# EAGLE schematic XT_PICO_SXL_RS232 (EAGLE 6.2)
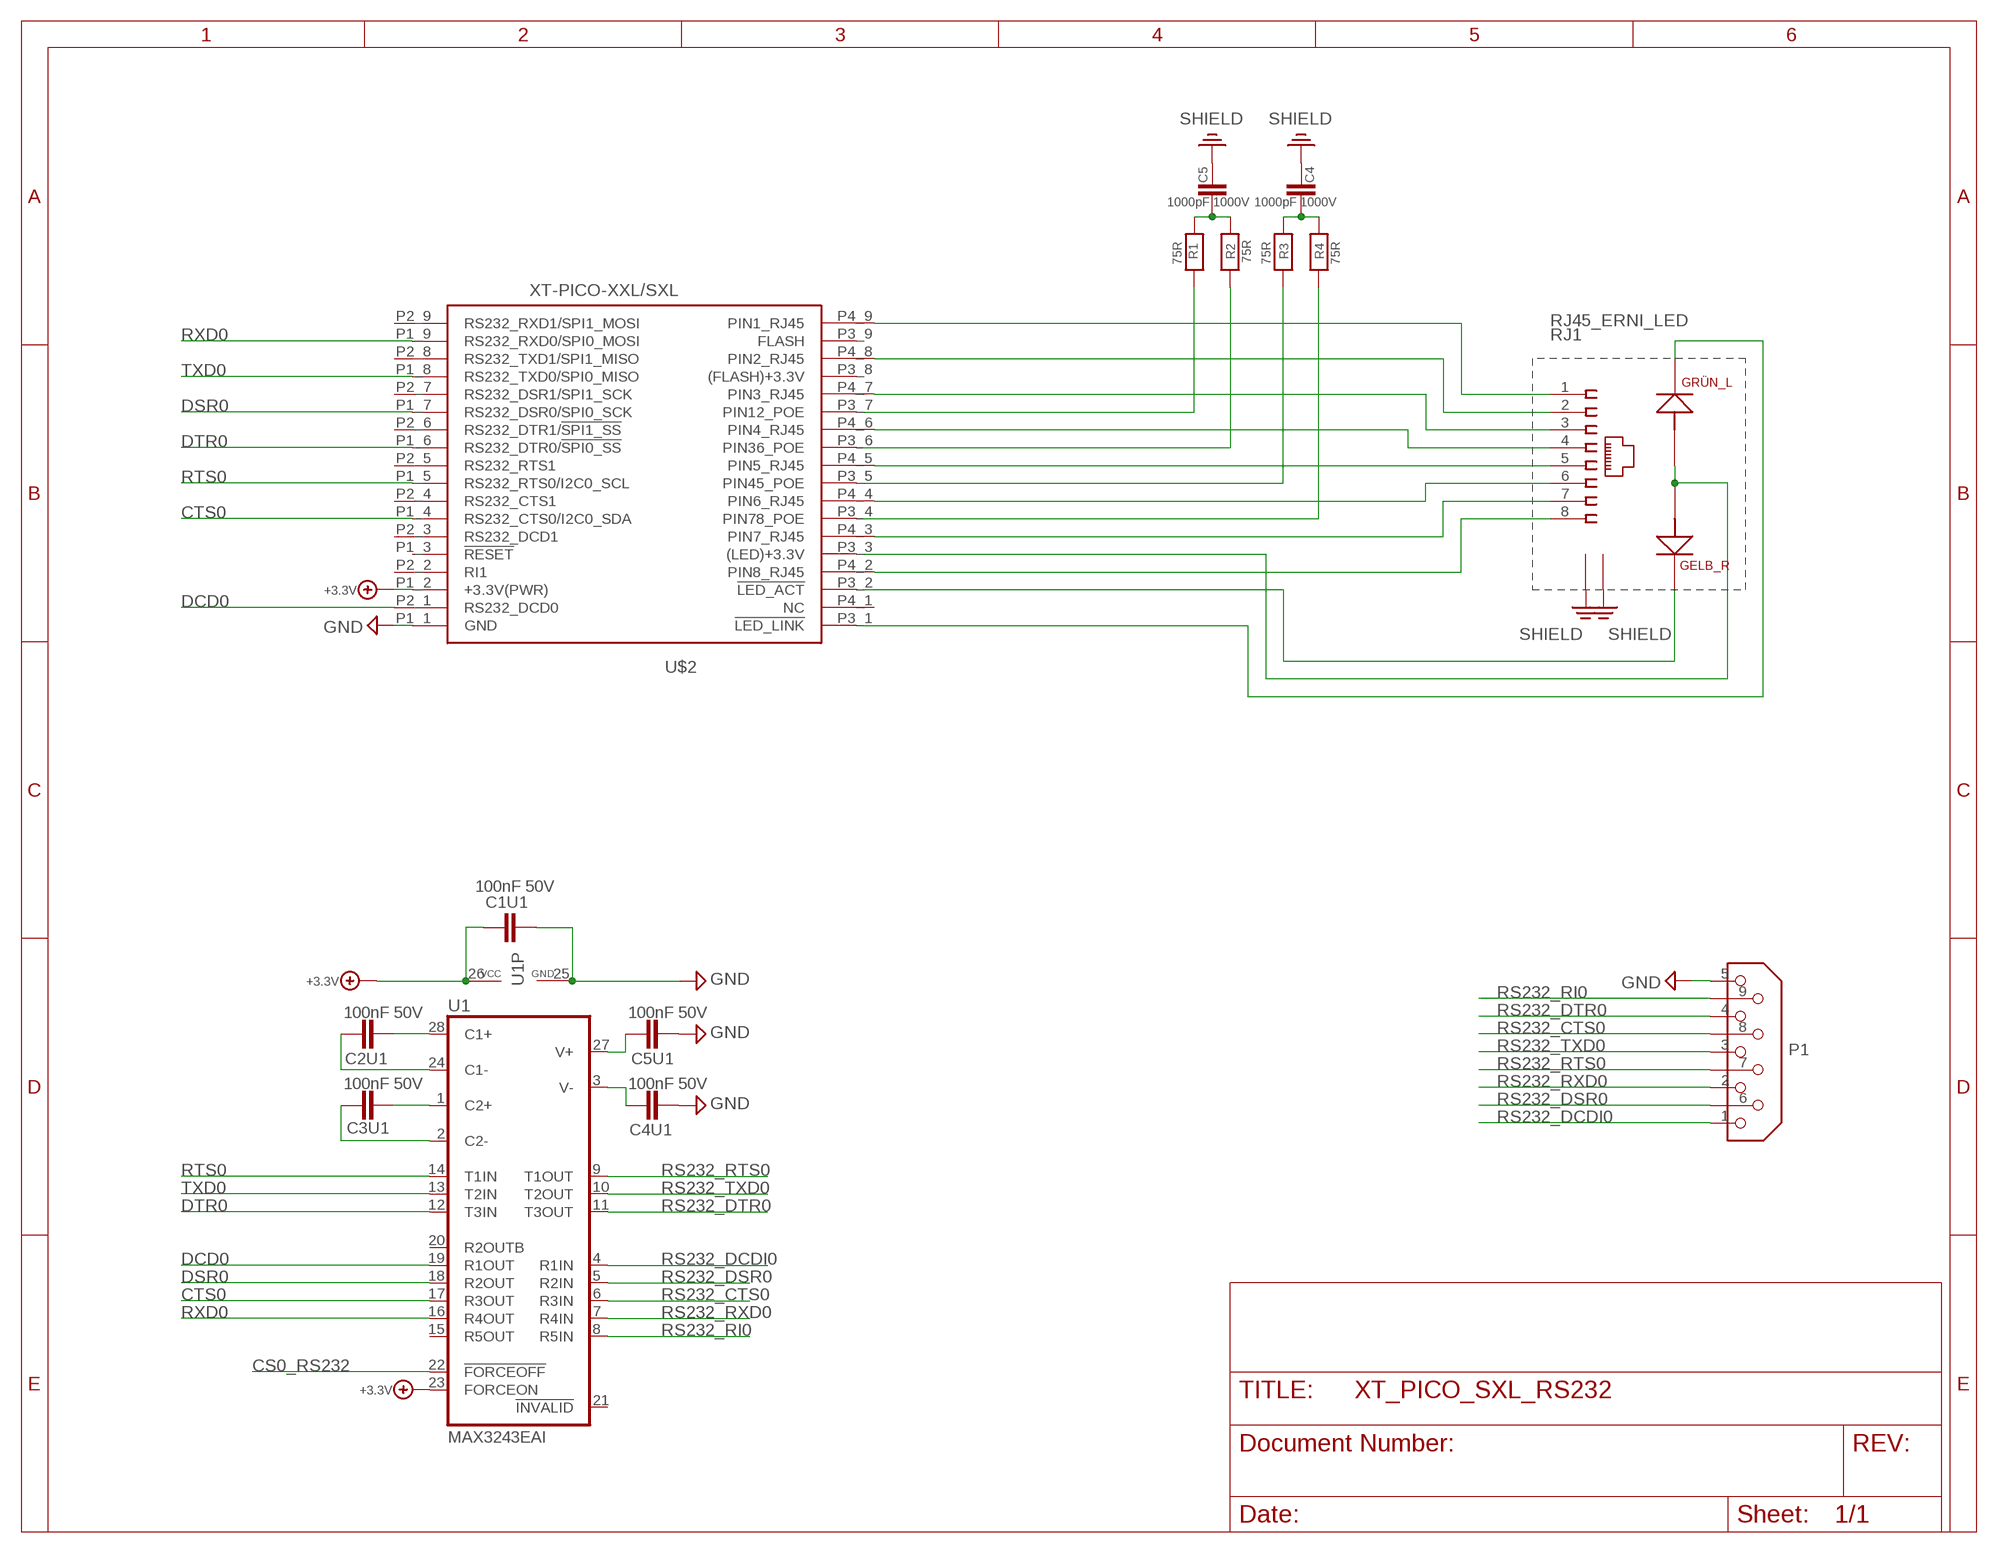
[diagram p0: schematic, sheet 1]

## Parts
C1U1  100nF 50V  CHIP-C-0603  [SMD-0603]
C2U1  100nF 50V  CHIP-C-0603  [SMD-0603]
C3U1  100nF 50V  CHIP-C-0603  [SMD-0603]
C4  1000pF 1000V  CHIP-C-1210  [SMD-1210]
C4U1  100nF 50V  CHIP-C-0603  [SMD-0603]
C5  1000pF 1000V  CHIP-C-1210  [SMD-1210]
C5U1  100nF 50V  CHIP-C-0603  [SMD-0603]
P1  DB9  [MSUB9-5]
R1  75R  CHIP-R-0603  [SMD-0603]
R2  75R  CHIP-R-0603  [SMD-0603]
R3  75R  CHIP-R-0603  [SMD-0603]
R4  75R  CHIP-R-0603  [SMD-0603]
RJ1  RJ45_ERNI_LED  [ORCAD_X_ERNI_RJ45_LED]
U1  MAX3243EAI  [SSOP28]
U$2  XT-PICO-XXL/SXL  [XT-PICO-XXL/SXL]

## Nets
+3.3V: C1U1.1 U1.23(FORCEON) U1.26(VCC) U$2.P1_2(+3.3V(PWR))
CS0_RS232: U1.22(!FORCEOFF)
CTS0: U1.17(R3OUT) U$2.P1_4(RS232_CTS0/I2C0_SDA)
DCD0: U1.19(R1OUT) U$2.P2_1(RS232_DCD0)
DSR0: U1.18(R2OUT) U$2.P1_7(RS232_DSR0/SPI0_SCK)
DTR0: U1.12(T3IN) U$2.P1_6(RS232_DTR0/!SPI0_SS!)
GND: C1U1.2 C4U1.2 C5U1.2 P1.5 U1.25(GND) U$2.P1_1(GND)
N$1: RJ1.4 U$2.P4_6(PIN4_RJ45)
N$2: RJ1.5 U$2.P4_5(PIN5_RJ45)
N$3: RJ1.7 U$2.P4_3(PIN7_RJ45)
N$4: R1.2 U$2.P3_7(PIN12_POE)
N$5: RJ1.8 U$2.P4_2(PIN8_RJ45)
N$6: R2.2 U$2.P3_6(PIN36_POE)
N$7: RJ1.1 U$2.P4_9(PIN1_RJ45)
N$8: RJ1.2 U$2.P4_8(PIN2_RJ45)
N$9: RJ1.3 U$2.P4_7(PIN3_RJ45)
N$10: R3.2 U$2.P3_5(PIN45_POE)
N$11: R4.2 U$2.P3_4(PIN78_POE)
N$12: RJ1.6 U$2.P4_4(PIN6_RJ45)
N$15: RJ1.A1 RJ1.A2 U$2.P3_3((LED)+3.3V)
N$16: RJ1.K1 U$2.P3_2(!LED_ACT)
N$17: RJ1.K2 U$2.P3_1(!LED_LINK)
N$19: C4.2 R3.1 R4.1
N$20: C5.1 R1.1 R2.1
N$22: C4U1.1 U1.3(V-)
N$23: C5U1.1 U1.27(V+)
N$24: C3U1.2 U1.1(C2+)
N$26: C2U1.2 U1.28(C1+)
N$27: C3U1.1 U1.2(C2-)
N$28: C2U1.1 U1.24(C1-)
PE: RJ1.9 RJ1.10 ; supply symbol labelled SHIELD
RS232_CTS0: P1.8 U1.6(R3IN)
RS232_DCDI0: P1.1 U1.4(R1IN)
RS232_DSR0: P1.6 U1.5(R2IN)
RS232_DTR0: P1.4 U1.11(T3OUT)
RS232_RI0: P1.9 U1.8(R5IN)
RS232_RTS0: P1.7 U1.9(T1OUT)
RS232_RXD0: P1.2 U1.7(R4IN)
RS232_TXD0: P1.3 U1.10(T2OUT)
RTS0: U1.14(T1IN) U$2.P1_5(RS232_RTS0/I2C0_SCL)
RXD0: U1.16(R4OUT) U$2.P1_9(RS232_RXD0/SPI0_MOSI)
SHIELD: C4.1 C5.2
TXD0: U1.13(T2IN) U$2.P1_8(RS232_TXD0/SPI0_MISO)
Unconnected: U1.15(R5OUT) U1.20(R2OUTB) U1.21(!INVALID) U$2.P1_3(!RESET) U$2.P2_2(RI1) U$2.P2_3(RS232_DCD1) U$2.P2_4(RS232_CTS1) U$2.P2_5(RS232_RTS1) U$2.P2_6(RS232_DTR1/!SPI1_SS!) U$2.P2_7(RS232_DSR1/SPI1_SCK) U$2.P2_8(RS232_TXD1/SPI1_MISO) U$2.P2_9(RS232_RXD1/SPI1_MOSI) U$2.P3_8((FLASH)+3.3V) U$2.P3_9(FLASH) U$2.P4_1(NC)

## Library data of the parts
C1U1 C2U1 C3U1 C4U1 C5U1 = mea-lib:CHIP-C-?: Chip capacitance
C4 C5 = XTMACRO:CHIP-C-?: Chip capacitance
P1 = XTMACRO:DB9
R1-R4 = XTMACRO:CHIP-R-?: Chip resistors
RJ1 = XTMACRO:RJ45_ERNI_LED
U1 = maxim:MAX3243*: RS-232 Transceivers with AutoShutdown 1µA Supply-Current, True +3V to +5.5V http://dbserv.maxim-ic.com/
U$2 = ak-devices:XT-PICO-XXL/SXL: AK-NORD XT-PICO-XXL/SXL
